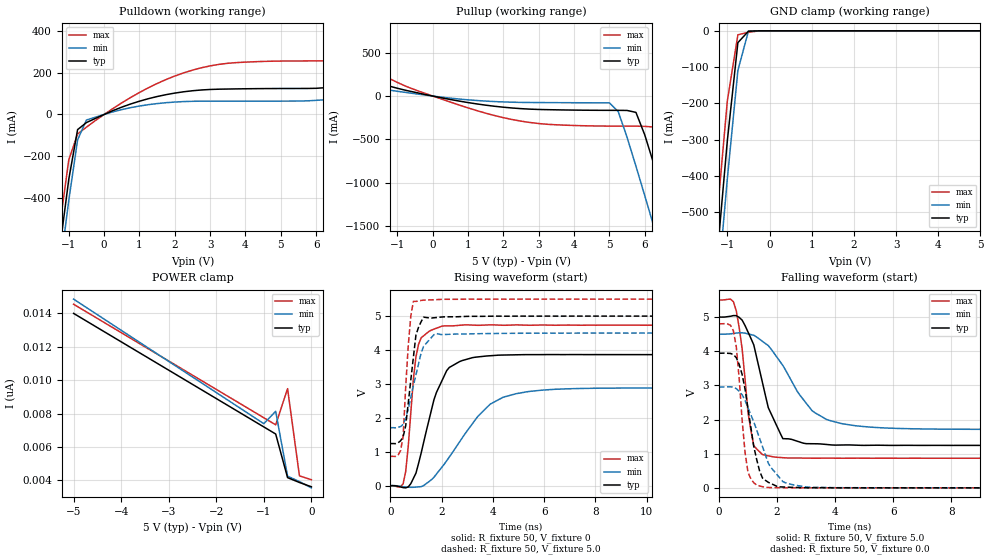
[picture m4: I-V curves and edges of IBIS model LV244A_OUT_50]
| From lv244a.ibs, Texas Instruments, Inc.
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|   Model LV244A_OUT_50
[Model]   LV244A_OUT_50
Model_type  3-state
Polarity   Non-Inverting
Enable   Active-Low
Vmeas = 2.5v
Cref = 15pf
| variable   typ   min   max
C_comp   5.8pf   4.35pf   7.25pf
[Temperature Range]   25   85   -40
[Voltage Range]   5.0   4.5   5.5
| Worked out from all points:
|   slope of the pulldown table from 0 to 0.75 V, typ, clamps not added: 14.9 ohm
|   slope of the pullup table from 0 to 0.75 V, typ, clamps not added: 12.9 ohm
|   GND clamp passes 1 mA (typ) near -0.46 V on its own axis
|   rising waveform, R_fixture 50, V_fixture 0: 20-80 % time 871ps typ, 1.72ns min, 327ps max; typ from 0 V to 3.86 V
|   falling waveform, R_fixture 50, V_fixture 5.0: 20-80 % time 726ps typ, 1.3ns min, 362ps max; typ from 5 V to 1.24 V
|   rising waveform, R_fixture 50, V_fixture 5.0: 20-80 % time 336ps typ, 515ps min, 227ps max; typ from 1.24 V to 5 V
|   falling waveform, R_fixture 50, V_fixture 0.0: 20-80 % time 474ps typ, 804ps min, 283ps max; typ from 3.94 V to 0 V
[Pulldown]
|   Voltage   I(typ)   I(min)   I(max)
-5V       -5.909A    -6.004A    -5.808A
-1.25V    -636.8mA   -741.3mA   -527.6mA
-1V       -311.1mA   -412.1mA   -218mA
-750mV    -72.57mA   -121.6mA   -93.4mA
-500mV    -38.76mA   -26.54mA   -60.93mA
250mV     18.47mA    12.63mA    28.54mA
1.5V      85.94mA    52.23mA    148.4mA
2.75V     117.3mA    63.71mA    223.6mA
3.75V     122.6mA    63.88mA    248.7mA
6V        125.5mA    67.63mA    256.7mA
6.75V     137.7mA    77.6mA     266.2mA
10V       220.2mA    122.3mA    416.3mA
[Pullup]
|   Voltage   I(typ)   I(min)   I(max)
-5V       413.4mA    223.7mA    779.9mA
-3.5V     335.8mA    190.4mA    616mA
-750mV    64.72mA    40.97mA    111.1mA
1.5V      -104.9mA   -57.9mA    -197.3mA
5V        -164.4mA   -78.35mA   -345.7mA
5.25V     -164.5mA   -179.5mA   -345.8mA
5.75V     -188mA     -806.5mA   -346.2mA
6.25V     -775.7mA   -1.492A    -355.9mA
6.5V      -1.117A    -1.839A    -497.7mA
6.75V     -1.462A    -2.188A    -820.3mA
7.25V     -2.161A    -2.89A     -1.508A
10V       -6.051A    -6.781A    -5.396A
[GND Clamp]
|   Voltage   I(typ)   I(min)   I(max)
-5V       -5.908A    -6.004A    -5.808A
-1.5V     -974.3mA   -1.079A    -862.7mA
-1.25V    -633mA     -739mA     -520.4mA
-1V       -303.2mA   -408.1mA   -193.1mA
-750mV    -32.52mA   -109.4mA   -10.91mA
-500mV    -1.18mA    -669.5uA   -3.99mA
-250mV    -36.94nA   -297.1nA   -155.5uA
5V        3.614nA    4.25nA     3.57nA
[POWER Clamp]
|   Voltage   I(typ)   I(min)   I(max)
-5V       14nA       14.86nA    14.55nA
-1V       7.2nA      7.395nA    7.75nA
-750mV    6.775nA    8.133nA    7.325nA
-500mV    4.161nA    4.25nA     9.493nA
-250mV    3.87nA     3.924nA    4.268nA
0V        3.614nA    3.548nA    4.036nA
[Ramp]
| variable   typ   min   max
dV/dt_r  2.3215E+00/8.2981E-10  1.7354E+00/1.7146E-09  2.8449E+00/3.2718E-10
dV/dt_f  2.2861E+00/7.0516E-10  1.6982E+00/1.2887E-09  2.5204E+00/4.3674E-10
R_load = 50
[Rising Waveform]
R_fixture = 50
V_fixture = 0
|   Time   V(typ)   V(min)   V(max)
0s        0V         0V         0V
400ps     -36.52mV   -15.73mV   -28.09mV
600ps     -63.83mV   -39mV      419.7mV
900ps     215mV      -46.82mV   3.14V
1.1ns     650.7mV    -34.11mV   4.163V
2ns       3.072V     534.1mV    4.701V
2.7ns     3.658V     1.291V     4.729V
3.9ns     3.832V     2.406V     4.743V
5.4ns     3.864V     2.777V     4.73V
25ns      3.863V     2.88V      4.731V
[Falling Waveform]
R_fixture = 50
V_fixture = 5.0
V_fixture_min = 4.5
V_fixture_max = 5.5
|   Time   V(typ)   V(min)   V(max)
0s        5V         4.5V       5.5V
600ps     5.041V     4.531V     5.173V
800ps     4.909V     4.54V      4.064V
1.1ns     4.378V     4.486V     1.684V
1.2ns     4.185V     4.466V     1.231V
1.5ns     3.076V     4.288V     972.8mV
2.2ns     1.44V      3.583V     882.9mV
3.2ns     1.291V     2.264V     867.8mV
4.7ns     1.25V      1.818V     868.2mV
25ns      1.242V     1.71V      866.1mV
[Rising Waveform]
R_fixture = 50
V_fixture = 5.0
V_fixture_min = 4.5
V_fixture_max = 5.5
|   Time   V(typ)   V(min)   V(max)
0s        1.242V     1.71V      866.1mV
300ps     1.264V     1.724V     898.1mV
500ps     1.441V     1.81V      1.449V
700ps     2.435V     2.261V     4.136V
800ps     3.123V     2.611V     5.003V
900ps     3.783V     2.946V     5.435V
1ns       4.443V     3.267V     5.433V
1.3ns     4.969V     4.111V     5.471V
1.8ns     4.958V     4.485V     5.486V
25ns      5V         4.5V       5.5V
[Falling Waveform]
R_fixture = 50
V_fixture = 0.0
|   Time   V(typ)   V(min)   V(max)
0s        3.942V     2.952V     4.803V
500ps     3.902V     2.947V     4.594V
600ps     3.808V     2.902V     4.118V
800ps     3.317V     2.726V     1.97V
1ns       2.327V     2.348V     457.4mV
1.3ns     830mV      1.693V     83.2mV
1.6ns     219.8mV    963.2mV    14.46mV
2.2ns     25.66mV    184.5mV    3.788mV
3.1ns     1.723mV    17.48mV    2.586mV
25ns      13.3uV     18.09uV    7.341uV
